| IBIS file abc.ibs created by s2ibis2 version 1.2
| North Carolina State University Electronics Research Laboratory  1995
[IBIS ver]   2.1
[File name]   idt70t6xx_208dr.ibs
[File Rev]   1.0
[Date]   12/19/2002
[Source]   Integrated Device Technology, Inc.
[Notes]   1.Temperatures: typ=25C, min=100C, max=0C 2.RRmp rates based
   on 50 ohm load.
[Disclaimer] Integrated Device Technology, Inc. ("IDT") hereby grants the
   user of this IBIS model a non-exclusive, nontransferable
   license to use this IBIS model under the following terms. The
   user is granted this license only to use the IBIS model and is
   not granted rights to sell, copy (except as needed to run the
   IBIS model), rent, lease or sub-license the IBIS model in
   whole or in part, or in modified form to anyone. The User may
   modify the IBIS model to suit its specific applications, but
   rights to derivative works and such modifications shall belong
   to IDT. This IBIS model is provided on an AS IS" basis and IDT
   makes absolutely no warranty with respect to the information
   contained herein. IDT DISCLAIMS AND CUSTOMER WAIVES ALL
   WARRANTIES, EXPRESS AND IMPLIED, INCLUDING WARRANTIES OF
   MERCHANTABILITY AND FITNESS FOR A PARTICULAR PURPOSE. THE
   ENTIRE RISK AS TO QUALITY AND PERFORMANCE IS WITH THE USER
   ACCORDINGLY, IN NO EVENT SHALL IDT BE LIABLE FOR ANY DIRECT OR
   INDIRECT DAMAGES, WHETHER IN CONTRACT OR TORT, INCLUDING ANY
   LOST PROFITS OR OTHER INCIDENTAL, CONSEQUENTIAL, EXEMPLARY, OR
   PUNITIVE DAMAGES ARISING OUT OF THE USE OR APPLICATION OF THE
   IBIS model. Further, IDT reserves the right to make changes
   without notice to any product herein to improve reliability,
   function, or design. IDT does not convey any license under
   patent rights or any other intellectual property rights,
   including those of third parties. IDT is not obligated to
   provide maintenance or support for the licensed IBIS model.
[Copyright]   Copyright 2001, Integrated Device Technology, Inc. all rights
   reserved
|   Component idt70t6xx_208dr
[Component]   idt70t6xx_208dr
[Manufacturer]   Integrated Device Technology
[Package]
| variable   typ   min   max
R_pkg   0.19600   0.19500   0.196000
L_pkg   13.1000nH   10.8200nH   15.36000nH
C_pkg   1.92000pF   1.90000pF   1.940000pF
| NOTE:
| The model_name inpad25, inpadzz25, inpadbs25, and iopad25 work for both 3.3v and 2.5v
| vddq.  When vddq is 3.3v, the model names are inpad33, inpadzz33, inpadbs33, and
| iopad33.  When vddq is 2.5v, the model names will be inpad25, inpadzz25, inpadbs25,
| and iopad25.
[Pin]  signal_name   model_name   R_pin   L_pin   C_pin
1   io19l   iopad25
2   io19r   iopad25
3   io20l   iopad25
4   io20r   iopad25
5   vddql   POWER
6   vss   GND
7   io21l   iopad25
8   io21r   iopad25
9   io22l   iopad25
10   io22r   iopad25
11   vddqr   POWER
12   vss   GND
13   io23l   iopad25
14   io23r   iopad25
15   io24l   iopad25
16   io24r   iopad25
17   vddql   POWER
18   vss   GND
19   io25l   iopad25
20   io25r   iopad25
21   io26l   iopad25
22   io26r   iopad25
23   vddqr   POWER
24   zzr   inpadzz25
25   vdd   POWER
26   vdd   POWER
27   vss   GND
28   vss   GND
29   vddql   POWER
30   vss   GND
31   io27r   iopad25
32   io27l   iopad25
33   io28r   iopad25
34   io28l   iopad25
35   vddqr   POWER
36   vss   GND
37   io29r   iopad25
38   io29l   iopad25
39   io30r   iopad25
40   io30l   iopad25
41   vddql   POWER
42   vss   GND
43   io31r   iopad25
44   io31l   iopad25
45   io32r   iopad25
46   io32l   iopad25
47   vddqr   POWER
48   vss   GND
49   io33r   iopad25
50   io33l   iopad25
51   io34r   iopad25
52   io34l   iopad25
53   vss   GND
54   vddql   POWER
55   io35r   iopad25
56   io35l   iopad25
57   vdd   POWER
58   tms   inpadbs25
59   tck   inpadbs25
60   trstb   inpadbs25
63   a17r   inpad25
64   a16r   inpad25
65   a15r   inpad25
66   a14r   inpad25
67   a13r   inpad25
68   a12r   inpad25
69   a11r   inpad25
70   a10r   inpad25
71   a9r   inpad25
72   a8r   inpad25
73   a7r   inpad25
74   be3rb   inpad25
75   be2rb   inpad25
76   be1rb   inpad25
77   be0rb   inpad25
78   ce1r   inpad25
79   ce0r   inpad25
80   vdd   POWER
81   vdd   POWER
82   vss   GND
83   vss   GND
84   semrb   inpad25
85   oerb   inpad25
86   rwrb   inpad25
87   busyrb   iopad25
88   intrb   iopad25
89   msb   inpad25
90   a6r   inpad25
91   a5r   inpad25
92   a4r   inpad25
93   a3r   inpad25
94   a2r   inpad25
95   a1r   inpad25
96   a0r   inpad25
97   vdd   POWER
98   vss   GND
99   vss   GND
100   optr   inpad25
101   io0l   iopad25
102   io0r   iopad25
103   vddql   POWER
104   vss   GND
105   io1l   iopad25
106   io1r   iopad25
107   io2l   iopad25
108   io2r   iopad25
109   vddqr   POWER
110   vss   GND
111   io3l   iopad25
112   io3r   iopad25
113   io4l   iopad25
114   io4r   iopad25
115   vddql   POWER
116   vss   GND
117   io5l   iopad25
118   io5r   iopad25
119   io6l   iopad25
120   io6r   iopad25
121   vddqr   POWER
122   vss   GND
123   io7l   iopad25
124   io7r   iopad25
125   io8l   iopad25
126   io8r   iopad25
127   vddql   POWER
128   zzl   inpadzz25
129   vss   GND
130   vss   GND
131   vdd   POWER
132   vdd   POWER
133   vddqr   POWER
134   vss   GND
135   io9r   iopad25
136   io9l   iopad25
137   io10r   iopad25
138   io10l   iopad25
139   vddql   POWER
140   vss   GND
141   io11r   iopad25
142   io11l   iopad25
143   io12r   iopad25
144   io12l   iopad25
145   vddqr   POWER
146   vss   GND
147   io13r   iopad25
148   io13l   iopad25
149   io14r   iopad25
150   io14l   iopad25
151   vddql   POWER
152   vss   GND
153   io15r   iopad25
154   io15l   iopad25
155   io16r   iopad25
156   io16l   iopad25
157   vss   GND
158   vddqr   POWER
159   io17r   iopad25
160   io17l   iopad25
161   optl   inpad25
162   vss   GND
163   vdd   POWER
164   vdd   POWER
165   a0l   inpad25
166   a1l   inpad25
167   a2l   inpad25
168   a3l   inpad25
169   a4l   inpad25
170   a5l   inpad25
171   a6l   inpad25
173   intlb   iopad25
174   busylb   iopad25
175   rwlb   inpad25
176   oelb   inpad25
177   semlb   inpad25
178   vss   GND
179   vss   GND
180   vdd   POWER
181   vdd   POWER
182   ce0lb   inpad25
183   ce1l   inpad25
184   be0lb   inpad25
185   be1lb   inpad25
186   be2lb   inpad25
187   be3lb   inpad25
188   a7l   inpad25
189   a8l   inpad25
190   a9l   inpad25
191   a10l   inpad25
192   a11l   inpad25
193   a12l   inpad25
194   a13l   inpad25
195   a14l   inpad25
196   a15l   inpad25
197   a16l   inpad25
198   a17l   inpad25
201   tdo   iopad25
202   tdi   inpadbs25
203   vdd   POWER
204   vss/test   GND
205   io18l   iopad25
206   io18r   iopad25
207   vddqr   POWER
208   vss   GND
|in   in   dummy_model
|oe   oe   dummy_model
| needed to give pads seperate POWER supply
[Pin Mapping] pulldown_ref   pullup_ref
1   vss   vddql
2   vss   vddqr
3   vss   vddql
4   vss   vddqr
5   nc   vddql
6   vss   nc
7   vss   vddql
8   vss   vddqr
9   vss   vddql
10   vss   vddqr
11   nc   vddqr
12   vss   nc
13   vss   vddql
14   vss   vddqr
15   vss   vddql
16   vss   vddqr
17   nc   vddql
18   vss   nc
19   vss   vddql
20   vss   vddqr
21   vss   vddql
22   vss   vddqr
23   nc   vddqr
24   vss   vdd
25   nc   vdd
26   nc   vdd
27   vss   nc
28   vss   nc
29   nc   vddql
30   vss   nc
31   vss   vddqr
32   vss   vddql
33   vss   vddqr
34   vss   vddql
35   nc   vddqr
36   vss   nc
37   vss   vddqr
38   vss   vddql
39   vss   vddqr
40   vss   vddql
41   nc   vddql
42   vss   nc
43   vss   vddqr
44   vss   vddql
45   vss   vddqr
46   vss   vddql
47   nc   vddqr
48   vss   nc
49   vss   vddqr
50   vss   vddql
51   vss   vddqr
52   vss   vddql
53   vss   nc
54   nc   vddql
55   vss   vddqr
56   vss   vddql
57   nc   vdd
58   vss   vdd
59   vss   vdd
60   vss   vdd
63   vss   vdd
64   vss   vdd
65   vss   vdd
66   vss   vdd
67   vss   vdd
68   vss   vdd
69   vss   vdd
70   vss   vdd
71   vss   vdd
72   vss   vdd
73   vss   vdd
74   vss   vdd
75   vss   vdd
76   vss   vdd
77   vss   vdd
78   vss   vdd
79   vss   vdd
80   nc   vdd
81   nc   vdd
82   vss   nc
83   vss   nc
84   vss   vdd
85   vss   vdd
86   vss   vdd
87   vss   vddqr
88   vss   vddqr
89   vss   vdd
90   vss   vdd
91   vss   vdd
92   vss   vdd
93   vss   vdd
94   vss   vdd
95   vss   vdd
96   vss   vdd
97   nc   vdd
98   vss   nc
99   vss   nc
100   vss   vdd
101   vss   vddql
102   vss   vddqr
103   nc   vddql
104   vss   nc
105   vss   vddql
106   vss   vddqr
107   vss   vddql
108   vss   vddqr
109   nc   vddqr
110   vss   nc
111   vss   vddql
112   vss   vddqr
113   vss   vddql
114   vss   vddqr
115   nc   vddql
116   vss   nc
117   vss   vddql
118   vss   vddqr
119   vss   vddql
120   vss   vddqr
121   nc   vddqr
122   vss   nc
123   vss   vddql
124   vss   vddqr
125   vss   vddql
126   vss   vddqr
127   nc   vddql
128   vss   vdd
129   vss   nc
130   vss   nc
131   nc   vdd
132   nc   vdd
133   nc   vddqr
134   vss   nc
135   vss   vddqr
136   vss   vddql
137   vss   vddqr
138   vss   vddql
139   nc   vddql
140   vss   nc
141   vss   vddqr
142   vss   vddql
143   vss   vddqr
144   vss   vddql
145   nc   vddqr
146   vss   nc
147   vss   vddqr
148   vss   vddql
149   vss   vddqr
150   vss   vddql
151   nc   vddql
152   vss   nc
153   vss   vddqr
154   vss   vddql
155   vss   vddqr
156   vss   vddql
157   vss   nc
158   nc   vddqr
159   vss   vddqr
160   vss   vddql
161   vss   vdd
162   vss   nc
163   nc   vdd
164   nc   vdd
165   vss   vdd
166   vss   vdd
167   vss   vdd
168   vss   vdd
169   vss   vdd
170   vss   vdd
171   vss   vdd
173   vss   vddql
174   vss   vddql
175   vss   vdd
176   vss   vdd
177   vss   vdd
178   vss   nc
179   vss   nc
180   nc   vdd
181   nc   vdd
182   vss   vdd
183   vss   vdd
184   vss   vdd
185   vss   vdd
186   vss   vdd
187   vss   vdd
188   vss   vdd
189   vss   vdd
190   vss   vdd
191   vss   vdd
192   vss   vdd
193   vss   vdd
194   vss   vdd
195   vss   vdd
196   vss   vdd
197   vss   vdd
198   vss   vdd
201   vss   vdd
202   vss   vdd
203   nc   vdd
204   vss/test   nc
205   vss   vddql
206   vss   vddqr
207   nc   vddqr
208   vss   nc
| Models and submodels in the file (8): inpad25 (Input), inpad33 (Input), inpadzz25 (Input), inpadzz33 (Input), inpadbs25 (Input), inpadbs33 (Input), iopad25 (I/O), iopad33 (I/O)
